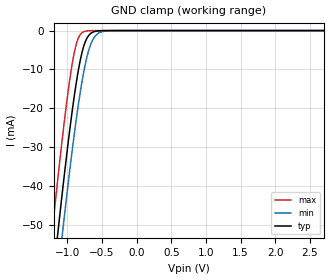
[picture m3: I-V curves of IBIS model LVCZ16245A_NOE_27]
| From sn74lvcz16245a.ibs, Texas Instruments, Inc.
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[Model]   LVCZ16245A_NOE_27
Model_type  Input
Vinl = 0.8
Vinh = 2
| variable   typ   min   max
C_comp   1.40pF   1.05pF   1.62pF
[Temperature Range]   40   100   -40
| Ambient temperature   25   85   -40
[Voltage range]   2.7   2.7   2.7
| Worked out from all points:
|   GND clamp passes 1 mA (typ) near -0.68 V on its own axis
[GND Clamp]
| LVCZ16245A_NOE_27
|   Voltage   I(typ)   I(min)   I(max)
-5V       -776.3mA   -784.3mA   -766.7mA
-1.24V    -69.32mA   -80.17mA   -55.39mA
-1.215V   -65.07mA   -75.94mA   -51.11mA
-1.14V    -52.55mA   -63.42mA   -38.55mA
-1.08V    -42.85mA   -53.67mA   -28.94mA
-1.06V    -39.7mA    -50.49mA   -25.86mA
-960mV    -24.78mA   -35.18mA   -11.94mA
-865mV    -12.71mA   -22.05mA   -3.093mA
-785mV    -5.383mA   -12.75mA   -501uA
-710mV    -1.72mA    -6.269mA   -68.68uA
-565mV    -106.8uA   -850.2uA   -1.322uA
2.7V      1.113nA    59.61nA    5.15pA
